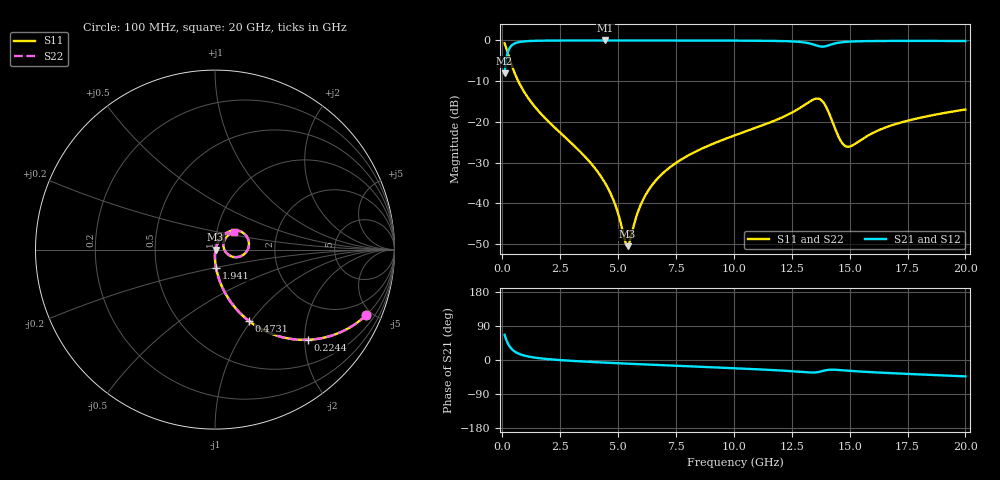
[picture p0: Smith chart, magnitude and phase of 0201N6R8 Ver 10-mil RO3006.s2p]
# GHz S MA R 50
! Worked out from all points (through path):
!   1601 points, 100 MHz to 20 GHz, reference 50 ohm
!   highest |S21| = -0.03 dB at 4.453 GHz (marker M1); lowest = -8.1 dB at 100 MHz (marker M2)
!   group delay of S21, straight-line fit = 7.57 ps
!   lowest |S11| = -50.5 dB at 5.411 GHz (marker M3), VSWR 1.01, Z = 50.3 - j0.0473 ohm
!   |S11| at or under -10 dB: 688.7 MHz to end of sweep
!   |S22| runs from -50.5 to -0.7 dB; largest |S21 - S12| = 0
!   S11 on the Smith chart (normalised r, x): 100 MHz: 0.99, -4.63; 224.4 MHz: 0.99, -2.06; 473.1 MHz: 0.99, -0.97; 1.941 GHz: 0.99, -0.21; 20 GHz: 1.20, +0.24
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0.1  0.919 -23.4  0.3938 66.6  0.3938 66.6  0.919 -23.4
0.224375  0.72 -44.3  0.6931 45.7  0.6931 45.7  0.72 -44.3
0.3363125  0.5684 -55.9  0.8218 34.0  0.8218 34.0  0.5684 -55.9
0.473125  0.4395 -64.6  0.8972 25.2  0.8972 25.2  0.4395 -64.6
0.920875  0.239 -77.5  0.9698 12.2  0.9698 12.2  0.239 -77.5
1.94075  0.1046 -86.5  0.9927 2.5  0.9927 2.5  0.1046 -86.5
3.420812  0.04154 -90.5  0.9967 -3.8  0.9967 -3.8  0.04154 -90.5
4.453125  0.01752 -88.1  0.997 -7.0  0.997 -7.0  0.01752 -88.1
4.876  0.009666 -81.2  0.997 -8.2  0.997 -8.2  0.009666 -81.2
5.298875  0.003483 -41.2  0.9969 -9.4  0.9969 -9.4  0.003483 -41.2
5.410812  0.002993 -9.0  0.9969 -9.7  0.9969 -9.7  0.002993 -9.0
6.032687  0.01042 60.8  0.9966 -11.4  0.9966 -11.4  0.01042 60.8
6.741625  0.02071 67.3  0.9962 -13.2  0.9962 -13.2  0.02071 67.3
8.01025  0.0385 67.7  0.9952 -16.5  0.9952 -16.5  0.0385 67.7
10.05  0.06855 63.7  0.9921 -21.8  0.9921 -21.8  0.06855 63.7
12.28875  0.1209 53.6  0.9763 -28.7  0.9763 -28.7  0.1209 53.6
13.37081  0.1841 29.4  0.9013 -33.1  0.9013 -33.1  0.1841 29.4
13.86831  0.1733 -5.1  0.8382 -28.5  0.8382 -28.5  0.1733 -5.1
14.56481  0.06211 -13.6  0.939 -26.6  0.939 -26.6  0.06211 -13.6
14.86331  0.04982 8.2  0.959 -28.0  0.959 -28.0  0.04982 8.2
16.69162  0.08831 47.3  0.9831 -34.4  0.9831 -34.4  0.08831 47.3
20  0.142 43.4  0.981 -43.2  0.981 -43.2  0.142 43.4
